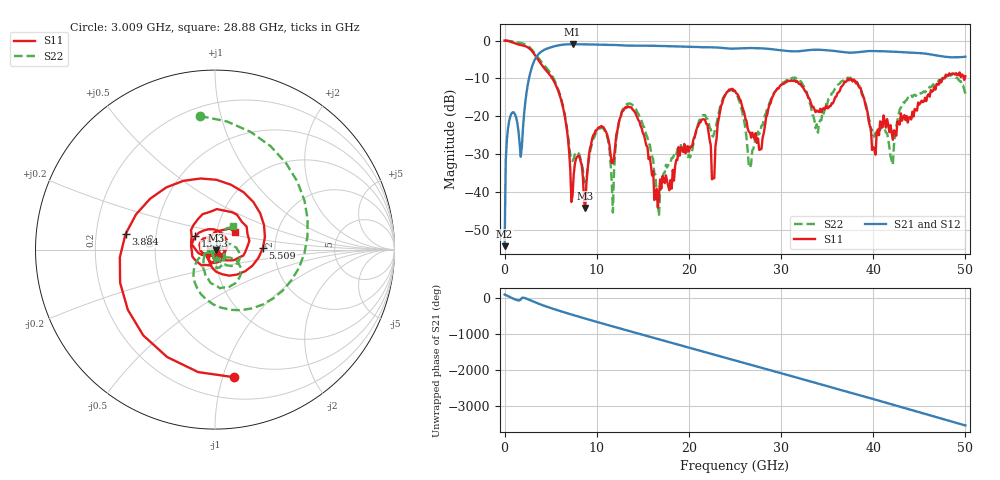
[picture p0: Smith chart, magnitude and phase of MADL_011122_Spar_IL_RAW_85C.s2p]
#	HZ	S	DB	R	50
!Frequency	S11 (dB)	S11-Ang	S21 (dB)	S21-Ang	S12 (dB)	S12-Ang	S22 (dB)	S22-Ang
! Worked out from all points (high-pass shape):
!   401 points, 10 MHz to 50 GHz, reference 50 ohm
!   highest |S21| = -0.96 dB at 7.384 GHz (marker M1); lowest = -54.4 dB at 10 MHz (marker M2)
!   |S21| within 3 dB of the highest: 3.561 GHz to 46.97 GHz (43.41 GHz wide, 172 % of centre)
!   lowest |S11| = -44.3 dB at 8.758 GHz (marker M3), VSWR 1.01, Z = 50.5 - j0.39 ohm
!   |S11| at or under -10 dB: 5.181 GHz to 47.58 GHz (42.4 GHz wide, 161 % of centre); 47.74235 GHz to 47.75177 GHz (9.416 MHz wide, 0.0197 % of centre); 49.83052 GHz to 49.92712 GHz (96.6 MHz wide, 0.194 % of centre)
!   |S22| runs from -46.4 to 0.0 dB; largest |S21 - S12| = 0.0072
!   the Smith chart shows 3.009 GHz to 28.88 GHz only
!   S11 on the Smith chart (normalised r, x): 3.009 GHz: 0.37, -1.09; 3.884 GHz: 0.33, +0.08; 5.509 GHz: 1.73, +0.03; 13.63 GHz: 0.79, +0.12; 28.88 GHz: 1.23, +0.25
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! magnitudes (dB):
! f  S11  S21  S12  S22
! 10 MHz  0.0  -54.4  -53.6  0.0
! 509.9 MHz  -0.2  -21.2  -21.2  -0.1
! 1.76 GHz  -1.2  -30.7  -30.7  -0.6
! 3.009 GHz  -2.9  -6.7  -6.7  -2.5
! 3.884 GHz  -5.9  -3.1  -3.1  -5.3
! 5.509 GHz  -11.5  -1.4  -1.5  -11.0
! 7.384 GHz  -40.9  -1.0  -1.0  -31.8
! 8.383 GHz  -33.0  -1.0  -1.0  -32.8
! 8.758 GHz  -44.3  -1.0  -1.0  -37.2
! 10.51 GHz  -22.6  -1.1  -1.1  -23.0
! 11.76 GHz  -32.4  -1.1  -1.2  -45.5
! 13.63 GHz  -17.6  -1.3  -1.4  -16.6
! 16.76 GHz  -40.9  -1.4  -1.4  -46.4
! 21.51 GHz  -20.8  -1.8  -1.8  -19.7
! 22.76 GHz  -36.4  -1.8  -1.8  -24.4
! 25 GHz  -13.2  -2.1  -2.1  -13.7
! 26.63 GHz  -24.3  -2.0  -2.0  -33.7
! 28.88 GHz  -16.5  -2.2  -2.3  -15.7
! 33.38 GHz  -17.5  -2.4  -2.5  -19.6
! 37.63 GHz  -10.1  -3.2  -3.2  -10.2
! 41.75 GHz  -24.2  -2.9  -2.9  -28.3
! 50 GHz  -9.4  -4.2  -4.2  -14.0
